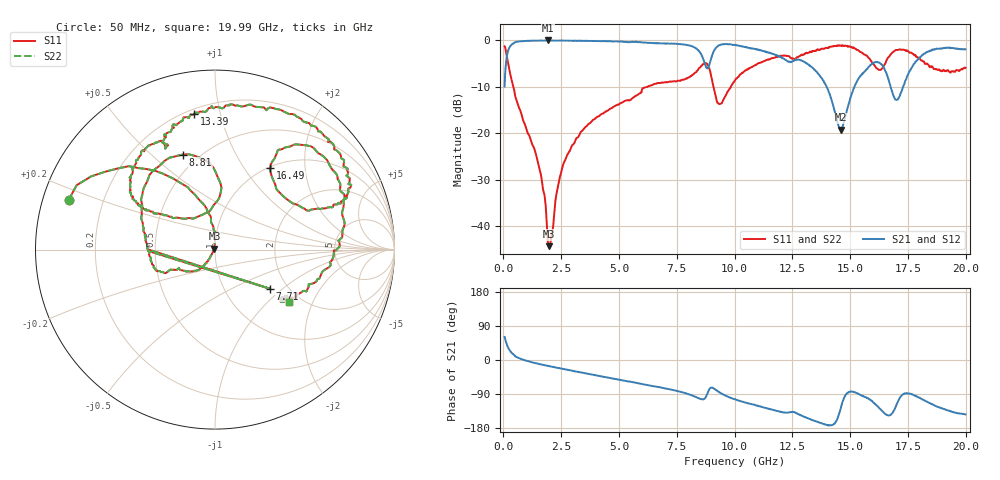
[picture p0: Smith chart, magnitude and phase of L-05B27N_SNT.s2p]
! Data Taken on a HP 8720C VNA using a shunt-through fixture with TRL* de-embedding
#	mhz	s	ma	r	50
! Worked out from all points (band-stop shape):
!   998 points, 50 MHz to 19.99 GHz, reference 50 ohm
!   highest |S21| = -0.02 dB at 1.93 GHz (marker M1); lowest = -19.2 dB at 14.59 GHz (marker M2)
!   |S21| within 3 dB of the highest: 162.6 MHz to 8.557 GHz (8.395 GHz wide, 193 % of centre); 9.046 GHz to 11.73 GHz (2.685 GHz wide, 25.8 % of centre)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
!   lowest |S11| = -44.3 dB at 1.97 GHz (marker M3), VSWR 1.01, Z = 49.7 + j0.534 ohm
!   |S11| at or under -10 dB: 426.9 MHz to 6.227 GHz (5.8 GHz wide, 174 % of centre); 9.09 GHz to 9.842 GHz (751.9 MHz wide, 7.94 % of centre)
!   |S22| runs from -44.3 to -1.1 dB; largest |S21 - S12| = 0
!   S11 on the Smith chart (normalised r, x): 50 MHz: 0.08, +0.16; 7.71 GHz: 1.62, -0.82; 8.81 GHz: 0.41, +0.63; 13.39 GHz: 0.23, +0.83; 16.49 GHz: 1.02, +1.33; 19.99 GHz: 1.74, -1.36
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50  0.8611 161.3  0.3193 60.8  0.3193 60.8  0.8611 161.3
510  0.25 103.0  0.9559 9.6  0.9559 9.6  0.25 103.0
1550  0.04272 89.7  0.9958 -10.8  0.9958 -10.8  0.04272 89.7
1930  0.00632 108.8  0.9975 -15.5  0.9975 -15.5  0.00632 108.8
1970  0.00607 117.8  0.9949 -16.0  0.9949 -16.0  0.00607 117.8
2550  0.04283 -124.7  0.9922 -23.3  0.9922 -23.3  0.04283 -124.7
3390  0.1052 -124.5  0.9872 -33.3  0.9872 -33.3  0.1052 -124.5
6710  0.3474 -160.2  0.9293 -71.4  0.9293 -71.4  0.3474 -160.2
7710  0.3744 -35.5  0.9083 -84.7  0.9083 -84.7  0.3744 -35.5
8810  0.5589 108.6  0.5002 -90.7  0.5002 -90.7  0.5589 108.6
9330  0.2061 109.9  0.8874 -84.7  0.8874 -84.7  0.2061 109.9
10030  0.3746 147.4  0.8885 -104.0  0.8885 -104.0  0.3746 147.4
13350  0.7651 100.3  0.515 -158.1  0.515 -158.1  0.7651 100.3
13390  0.7649 98.8  0.5026 -158.8  0.5026 -158.8  0.7649 98.8
14590  0.8776 46.2  0.1092 -128.3  0.1092 -128.3  0.8776 46.2
15710  0.6872 20.3  0.4876 -99.3  0.4876 -99.3  0.6872 20.3
16490  0.5489 55.7  0.4929 -140.7  0.4929 -140.7  0.5489 55.7
16670  0.6624 57.3  0.373 -146.4  0.373 -146.4  0.6624 57.3
17030  0.7883 44.9  0.2286 -115.2  0.2286 -115.2  0.7883 44.9
17570  0.7375 16.3  0.4633 -89.1  0.4633 -89.1  0.7375 16.3
18350  0.5606 -24.6  0.7537 -110.7  0.7537 -110.7  0.5606 -24.6
19990  0.5065 -35.1  0.8011 -143.6  0.8011 -143.6  0.5065 -35.1
